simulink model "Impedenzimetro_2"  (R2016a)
settings: Solver=VariableStepAuto  StartTime=0.0  StopTime=Tsim  RelTol=1e-3
undefined symbols (not defined in the file): C, f, Gain, L, R1, R2, Tsample, Vpeak, Vpeak_QAM, w
libraries: powerlib x7

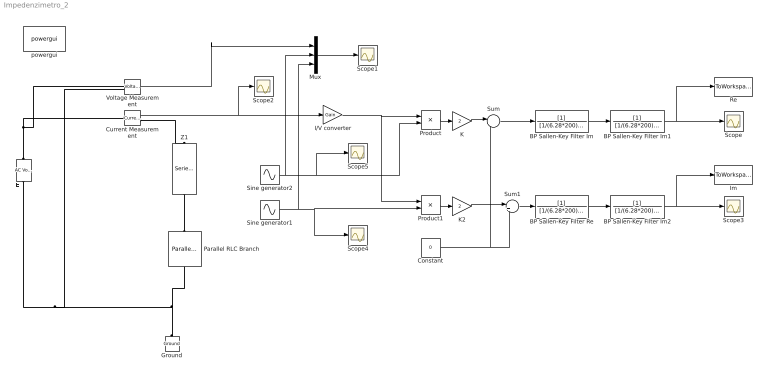
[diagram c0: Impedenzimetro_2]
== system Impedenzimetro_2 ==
  BP Sallen-Key Filter Im : TransferFcn  Denominator=[1/(6.28*200) 1]
  BP Sallen-Key Filter Im1 : TransferFcn  Denominator=[1/(6.28*200) 1]
  BP Sallen-Key Filter Im2 : TransferFcn  Denominator=[1/(6.28*200) 1]
  BP Sallen-Key Filter Re : TransferFcn  Denominator=[1/(6.28*200) 1]
  Constant : Constant  Value=0
  Current Measurement : powerlib/Measurements/Current Measurement  PhasorSimulation=off  OutputType=Complex  PSBequivalent=0
  E : powerlib/Electrical Sources/AC Voltage Source  Amplitude=Vpeak  Phase=0  Frequency=f  SampleTime=0  Measurements=None  BusType=swing  Pref=10e3  Qref=0  Qmin=-inf  Qmax=+inf
  Ground : powerlib/Elements/Ground  LConnTagsString=a
  I/V converter : Gain  Gain=Gain
  Im : ToWorkspace  VariableName=Im  SampleTime=-1
  K : Gain  Gain=2
  K2 : Gain  Gain=2
  Mux : Mux  Inputs=3
  Parallel RLC Branch : powerlib/Elements/Parallel RLC Branch  LConnTagsString=a  RConnTagsString=__new0  BranchType=RC  Resistance=R2  Inductance=L  SetiL0=off  InitialCurrent=0  Capacitance=C  Setx0=off  InitialVoltage=0  Measurements=None
  Product : Product
  Product1 : Product
  Re : ToWorkspace  VariableName=Re  SampleTime=-1
  Scope{,1..5} (6 alike) : Scope
  Sine generator1 : Sin  Amplitude=Vpeak_QAM  Frequency=w  Phase=(3.14/2)  SampleTime=0
  Sine generator2 : Sin  Amplitude=Vpeak_QAM  Frequency=w  SampleTime=0
  Sum : Sum  Inputs=|++
  Sum1 : Sum  Inputs=|++
  Voltage Measurement : powerlib/Measurements/Voltage Measurement  PhasorSimulation=off  OutputType=Complex  PSBequivalent=0
  Z1 : powerlib/Elements/Series RLC Branch  LConnTagsString=__new0  RConnTagsString=__new0  BranchType=R  Resistance=R1  Inductance=L  SetiL0=off  InitialCurrent=0  Capacitance=C  Setx0=off  InitialVoltage=0  Measurements=None
  powergui : powerlib/powergui  Priority=1  SimulationMode=Discrete  SolverType=Backward Euler  SampleTime=Tsample  frequency=f  SPID=off  DisableSnubberDevices=off  DisableRonSwitches=off  DisableVfSwitches=off  SwTol=0  DisplayEquations=off  Interpol=off  ExternalGateDelay=off  methode=off  Ts=10  FunctionMessages=off  echomessages=off  HookPort=off  EnableUseOfTLC=off  x0status=blocks  frequencyindice=200000  Pbase=100e6  ErrMax=1e-4  Iterations=50  UnitsV=kV  UnitsW=MW  buscounter=0  RestoreLinks=warning  ResistiveCurrentMeasurement=off  Frange=[0:2:500]  Ylog=off  Xlog=on  ShowGrid=off  save=off  variable=ZData  structure=0  ZoomFFT=off  StartTime=0.0  cycles=1  DisplayStyle=1  fundamental=60  FreqAxis=off  MaxFrequency=1000  frequencyindicesteady=1  RmsSteady=1  display=off
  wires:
  Current Measurement/1 -> Scope2/1, I/V converter/1
  I/V converter/1 -> Product1/1, Product/1
  BP Sallen-Key Filter Im/1 -> BP Sallen-Key Filter Im1/1
  Sine generator1/1 -> Mux/3, Scope4/1, Product1/2
  BP Sallen-Key Filter Re/1 -> BP Sallen-Key Filter Im2/1
  Sine generator2/1 -> Mux/2, Scope5/1, Product/2
  Mux/1 -> Scope1/1
  Voltage Measurement/1 -> Mux/1
  Product/1 -> K/1
  Sum/1 -> BP Sallen-Key Filter Im/1
  Product1/1 -> K2/1
  Sum1/1 -> BP Sallen-Key Filter Re/1
  Constant/1 -> Sum1/2, Sum/2
  K/1 -> Sum/1
  K2/1 -> Sum1/1
  BP Sallen-Key Filter Im1/1 -> Re/1, Scope/1
  BP Sallen-Key Filter Im2/1 -> Im/1, Scope3/1
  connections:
  E/RConn1 -- Voltage Measurement/LConn1 -- Current Measurement/LConn1
  Current Measurement/RConn1 -- Z1/LConn1
  Ground/LConn1 -- Parallel RLC Branch/RConn1 -- Voltage Measurement/LConn2 -- E/LConn1
  Parallel RLC Branch/LConn1 -- Z1/RConn1
